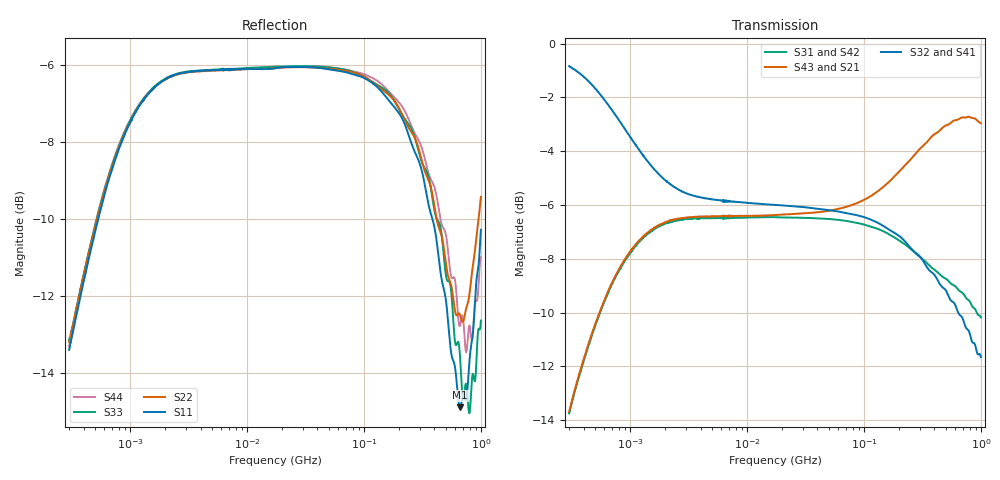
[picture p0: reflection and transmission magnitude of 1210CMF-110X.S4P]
!s-Parameter Generated by FASTRON Sdn. Bhd.
!FASTRON P/N : 1210CMF-110X
!Keysight Technologies: E5071C_MY46733604_B.14.02
!Date: Mon Mar 09 14:25:06 2026
!Version  :Rev00  Mon Mar 09 14:25:06 2026
!Data & Calibration Information:
!Freq	S11:SOLT4(ON)	S12:SOLT4(ON)	S13:SOLT4(ON)	S14:SOLT4(ON)
!	S21:SOLT4(ON)	S22:SOLT4(ON)	S23:SOLT4(ON)	S24:SOLT4(ON)
!	S31:SOLT4(ON)	S32:SOLT4(ON)	S33:SOLT4(ON)	S34:SOLT4(ON)
!	S41:SOLT4(ON)	S42:SOLT4(ON)	S43:SOLT4(ON)	S44:SOLT4(ON)
!PortZ  Port1:50+j0  Port2:50+j0  Port3:50+j0  Port4:50+j0
!When reading reference impedance value at option line is always used.
! Remarks : This data is being provided solely for informational purposes.
# Hz S dB R 50
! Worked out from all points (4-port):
!   1601 points, 300 kHz to 1 GHz, reference 50 ohm
!   strongest paths, dB at 300 kHz, 2.303 MHz, 17.55 MHz, 132.8 MHz, 1 GHz:
!     S32: -0.8, -5.3, -6.0, -6.7, -11.7
!     S41: -0.7, -5.3, -6.0, -6.7, -11.6
!     S43: -13.7, -6.5, -6.4, -5.5, -3.0
!     S21: -13.7, -6.6, -6.4, -5.4, -3.4
!     S31: -13.7, -6.6, -6.5, -6.9, -10.2
!     S42: -13.7, -6.6, -6.5, -6.9, -10.7
!   lowest |S11| = -14.9 dB at 663.3 MHz (marker M1), VSWR 1.44, Z = 71.8 - j2.4 ohm
!   |S11| at or under -10 dB: start of sweep to 533.3 kHz; 384.7 MHz to end of sweep
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300000  -13.40 57.5  -13.76 64.0  -13.76 -116.1  -0.77 -12.0
        -13.72 63.8  -13.19 54.5  -0.84 -12.1  -13.86 -116.0
        -13.74 -116.2  -0.84 -12.1  -13.15 54.5  -13.83 64.2
        -0.66 -12.6  -13.73 -116.3  -13.69 63.8  -13.31 59.8
1393703  -6.79 23.7  -7.05 24.5  -7.04 -156.0  -4.28 -18.3
         -7.07 24.5  -6.78 22.7  -4.33 -17.7  -7.09 -155.9
         -7.09 -156.0  -4.35 -17.7  -6.77 22.7  -7.04 24.5
         -4.31 -18.2  -7.11 -155.9  -7.03 24.6  -6.77 23.5
5596854  -6.13 5.2  -6.45 6.5  -6.45 -175.3  -5.82 -7.0
         -6.46 6.5  -6.14 5.0  -5.80 -6.8  -6.49 -175.2
         -6.49 -175.3  -5.82 -6.8  -6.12 4.9  -6.45 6.5
         -5.82 -7.0  -6.48 -175.1  -6.42 6.5  -6.14 5.3
4.011479e7  -6.07 -4.9  -6.29 5.1  -6.48 172.8  -6.15 -8.5
            -6.30 5.1  -6.07 -4.5  -6.13 -8.8  -6.53 173.6
            -6.50 172.8  -6.14 -8.9  -6.04 -5.1  -6.30 5.0
            -6.14 -8.5  -6.51 173.5  -6.27 4.9  -6.04 -3.8
2.209589e8  -7.51 -27.3  -4.47 12.1  -7.43 140.5  -7.31 -35.0
            -4.48 12.1  -7.41 -24.2  -7.31 -36.3  -7.46 145.1
            -7.44 140.6  -7.32 -36.3  -7.38 -28.3  -4.58 12.7
            -7.31 -34.9  -7.46 145.2  -4.56 12.6  -7.17 -22.1
6.63301e8  -14.90 -5.2  -2.77 0.3  -9.21 86.7  -9.81 -87.7
           -2.78 0.4  -12.49 -1.0  -10.10 -87.1  -9.35 95.3
           -9.21 86.8  -10.10 -87.2  -13.58 -15.5  -2.80 4.1
           -9.85 -87.7  -9.35 95.3  -2.78 4.0  -12.77 -11.3
1e9  -10.28 42.0  -3.35 -8.8  -10.18 54.6  -11.60 -126.0
     -3.37 -8.6  -9.43 39.3  -11.67 -124.8  -10.74 63.6
     -10.18 54.6  -11.65 -125.0  -12.64 40.9  -2.99 -3.8
     -11.63 -126.4  -10.75 63.6  -2.96 -3.6  -10.99 33.0
